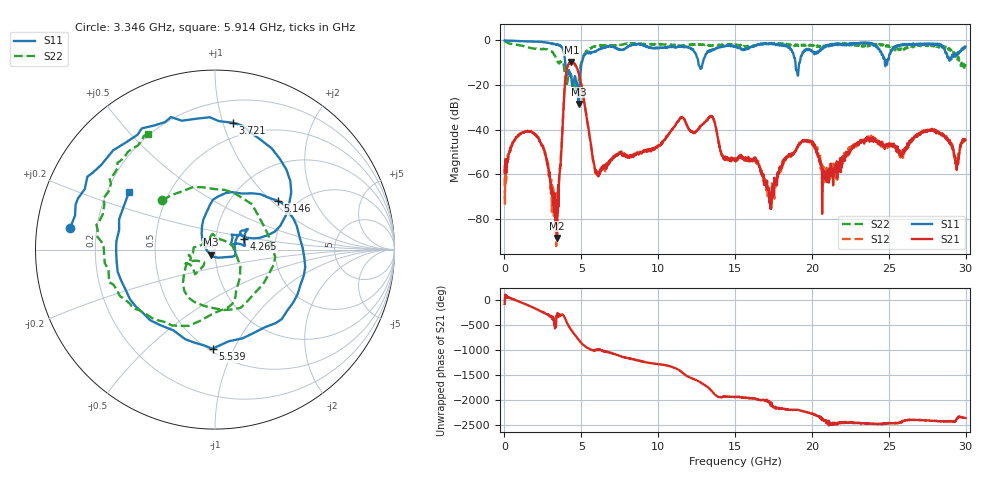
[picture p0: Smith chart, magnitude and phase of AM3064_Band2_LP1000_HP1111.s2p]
# Hz S DB R 50.0
!freq dBS11 angS11 dBS21 angS21 dBS12 angS12 dBS22 angS22
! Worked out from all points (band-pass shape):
!   1600 points, 10 MHz to 29.98 GHz, reference 50 ohm
!   highest |S21| = -9.62 dB at 4.359 GHz (marker M1); lowest = -88.5 dB at 3.421 GHz (marker M2)
!   |S21| within 3 dB of the highest: 4.06 GHz to 4.731 GHz (670.7 MHz wide, 15.3 % of centre)
!   lowest |S11| = -28.5 dB at 4.827 GHz (marker M3), VSWR 1.08, Z = 47.5 - j2.73 ohm
!   |S11| at or under -10 dB: 3.958 GHz to 5.03 GHz (1.072 GHz wide, 23.9 % of centre); 12.62 GHz to 12.9 GHz (280.6 MHz wide, 2.2 % of centre); 18.93 GHz to 19.18 GHz (256.3 MHz wide, 1.35 % of centre)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
!   |S22| runs from -23.9 to -0.2 dB; largest |S21 - S12| = 0.0095
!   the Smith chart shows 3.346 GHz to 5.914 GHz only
!   S11 on the Smith chart (normalised r, x): 3.346 GHz: 0.10, +0.07; 3.721 GHz: 0.37, +1.08; 4.265 GHz: 1.37, +0.16; 5.146 GHz: 1.63, +1.10; 5.539 GHz: 0.52, -0.83; 5.914 GHz: 0.29, +0.28
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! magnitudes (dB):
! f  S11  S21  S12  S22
! 10 MHz  0.0  -58.2  -55.9  -0.2
! 1.866 GHz  -0.6  -41.5  -41.4  -3.6
! 3.346 GHz  -1.8  -76.6  -76.2  -7.9
! 3.421 GHz  -1.9  -88.5  -69.0  -9.0
! 3.721 GHz  -2.9  -46.6  -46.9  -9.0
! 3.984 GHz  -11.8  -16.0  -16.0  -19.3
! 4.265 GHz  -15.3  -10.0  -9.9  -15.8
! 4.359 GHz  -17.5  -9.6  -9.6  -16.2
! 4.827 GHz  -28.5  -14.5  -14.5  -18.0
! 5.015 GHz  -10.5  -20.6  -20.4  -9.6
! 5.146 GHz  -7.0  -25.9  -25.9  -6.8
! 5.539 GHz  -5.1  -42.9  -43.0  -3.6
! 5.914 GHz  -4.8  -59.1  -59.3  -2.6
! 10 GHz  -3.4  -47.2  -47.1  -1.8
! 13.43 GHz  -4.6  -33.7  -33.7  -2.3
! 15 GHz  -2.6  -53.7  -53.3  -1.9
! 17.35 GHz  -1.4  -75.3  -69.0  -1.1
! 19.99 GHz  -4.6  -45.5  -45.9  -2.0
! 20.8 GHz  -2.7  -59.9  -59.9  -2.5
! 25 GHz  -8.1  -47.4  -46.1  -2.3
! 29.4 GHz  -6.2  -56.4  -56.6  -6.8
! 29.98 GHz  -2.7  -44.5  -45.1  -10.5
